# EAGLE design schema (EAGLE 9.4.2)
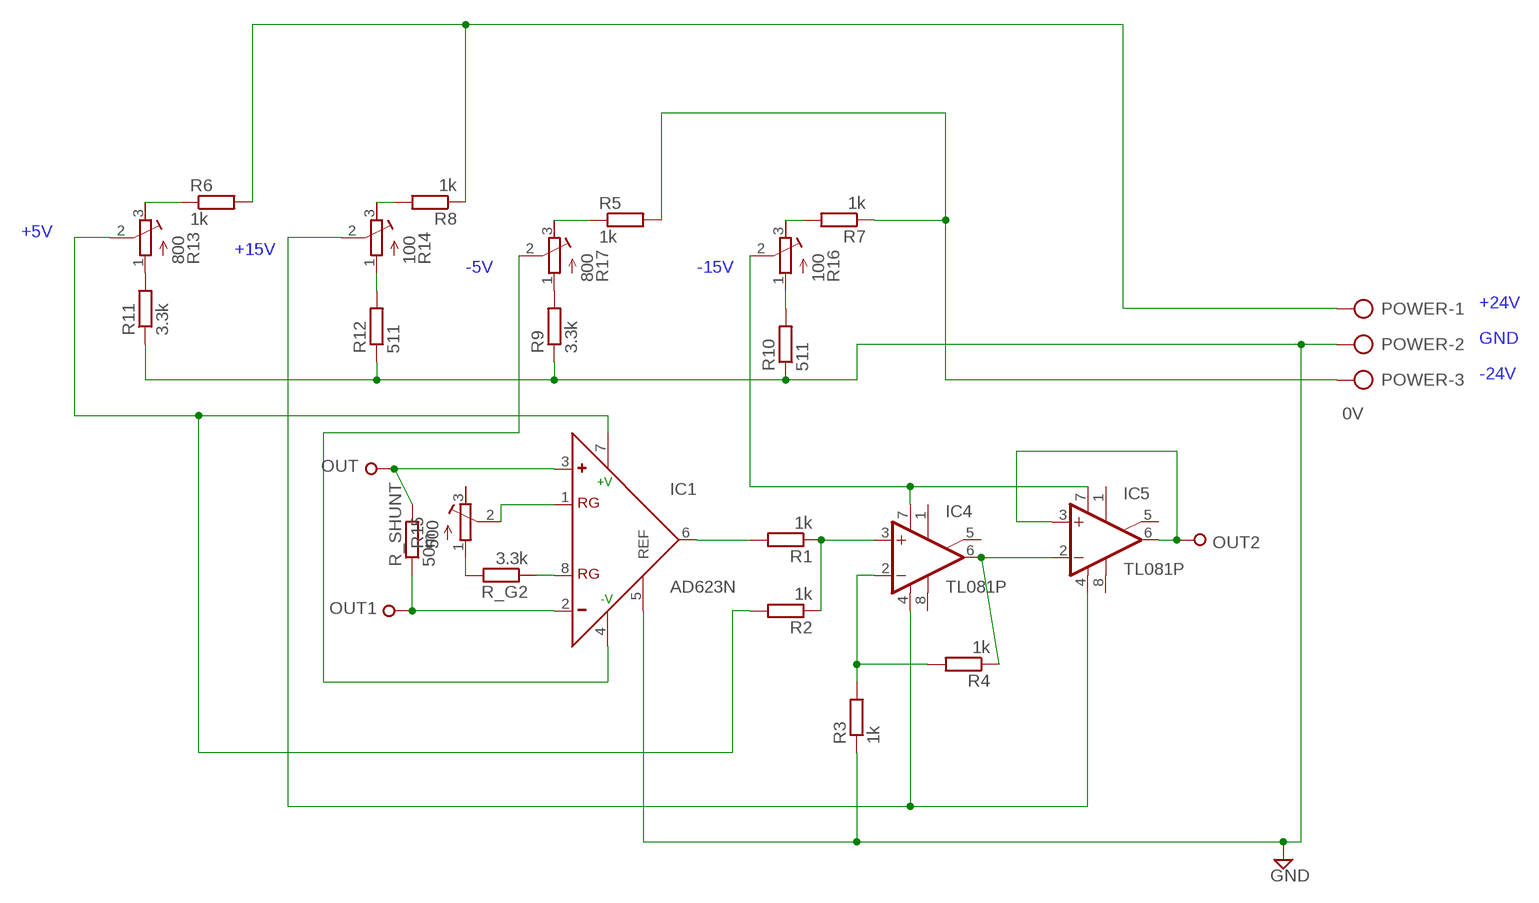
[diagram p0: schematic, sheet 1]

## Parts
IC1  AD623N  [DIL08]
IC4  TL081P  [DIL08]
IC5  TL081P  [DIL08]
OUT  SPECIAL_DRILL_0.2500  [PAD_0.2500]
OUT1  SPECIAL_DRILL_0.2500  [PAD_0.2500]
OUT2  SPECIAL_DRILL_0.2500  [PAD_0.2500]
POWER  0V  AK500/3-H  [AK500/3-H]
R1  1k  R-EU_0411/15  [0411/15]
R2  1k  R-EU_0411/15  [0411/15]
R3  1k  R-EU_0411/15  [0411/15]
R4  1k  R-EU_0411/15  [0411/15]
R5  1k  R-EU_0411/15  [0411/15]
R6  1k  R-EU_0411/15  [0411/15]
R7  1k  R-EU_0411/15  [0411/15]
R8  1k  R-EU_0411/15  [0411/15]
R9  3.3k  R-EU_0411/15  [0411/15]
R10  511  R-EU_0411/15  [0411/15]
R11  3.3k  R-EU_0411/15  [0411/15]
R12  511  R-EU_0411/15  [0411/15]
R13  800  R-TRIMM64X  [RTRIM64X]
R14  100  R-TRIMM64X  [RTRIM64X]
R15  500  R-TRIMM64X  [RTRIM64X]
R16  100  R-TRIMM64X  [RTRIM64X]
R17  800  R-TRIMM64X  [RTRIM64X]
R_G2  3.3k  R-EU_0411/15  [0411/15]
R_SHUNT  50m  R-EU_0309/12  [0309/12]

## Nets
GND: IC1.5(REF) POWER.2 R3.1 R9.1 R10.1 R11.1 R12.1
N$1: IC1.6(OUT) R1.2
N$2: IC4.2(-IN) R3.2 R4.2
N$3: IC4.3(+IN) R1.1 R2.1
N$4: IC4.6(OUT) IC5.2(-IN) R4.1
N$5: R15.1(A) R_G2.2
N$6: IC1.1(RG) R15.2(S)
N$7: IC1.8(RG) R_G2.1
N$8: IC1.2(-) OUT1.1 R_SHUNT.1
N$9: IC1.3(+) OUT.1 R_SHUNT.2
N$10: IC5.3(+IN) IC5.6(OUT) OUT2.1
N$11: R7.2 R16.3(E)
N$12: R5.1 R17.3(E)
N$13: R9.2 R17.1(A)
N$14: R10.2 R16.1(A)
N$15: R8.2 R14.3(E)
N$16: R6.1 R13.3(E)
N$17: R11.2 R13.1(A)
N$18: R12.2 R14.1(A)
N$19: POWER.1 R6.2 R8.1
N$20: POWER.3 R5.2 R7.1
N$22: IC4.7(V+) IC5.7(V+) R16.2(S)
N$23: IC1.4(-V) R17.2(S)
N$24: IC4.4(V-) IC5.4(V-) R14.2(S)
N$25: IC1.7(+V) R2.2 R13.2(S)
Unconnected: IC4.1(ON1) IC4.5(ON2) IC4.8(OPT) IC5.1(ON1) IC5.5(ON2) IC5.8(OPT) R15.3(E)

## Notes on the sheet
- +5V
- +15V
- -5V | -15V
- +24V
- GND
- -24V

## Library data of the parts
IC1 = analog-devices:AD623: Single-Supply, Rail-to-Rail, Low Cost Instrumentation Amplifier Source: http://www.analog.com/static/imported-files/data_sheets/AD623.pdf; MF: ALTERA CORPORATION; MPN: AD623ANZ; OC_FARNELL: 9603700; OC_NEWARK: 59K4402
IC4 IC5 = linear:TL081: OP AMP
OUT OUT1 OUT2 = special-drill:SPECIAL_DRILL_: Special drills
POWER = con-ptr500:AK500/3-H: CONNECTOR Aug. 2004 / PTR Meßtechnik: Die Bezeichnung der Serie AK505 wurde geändert. Es handelt sich hierbei um AK500 in horizontaler Ausführung.; OC_FARNELL: unknown; OC_NEWARK: unknown
R1-R12 R_G2 R_SHUNT = rcl:R-EU_: RESISTOR, European symbol; SPICEPREFIX: R
R13-R17 = rcl:R-TRIMM: Trimm resistor; SPICEMODEL: X; SPICEPREFIXL: POT

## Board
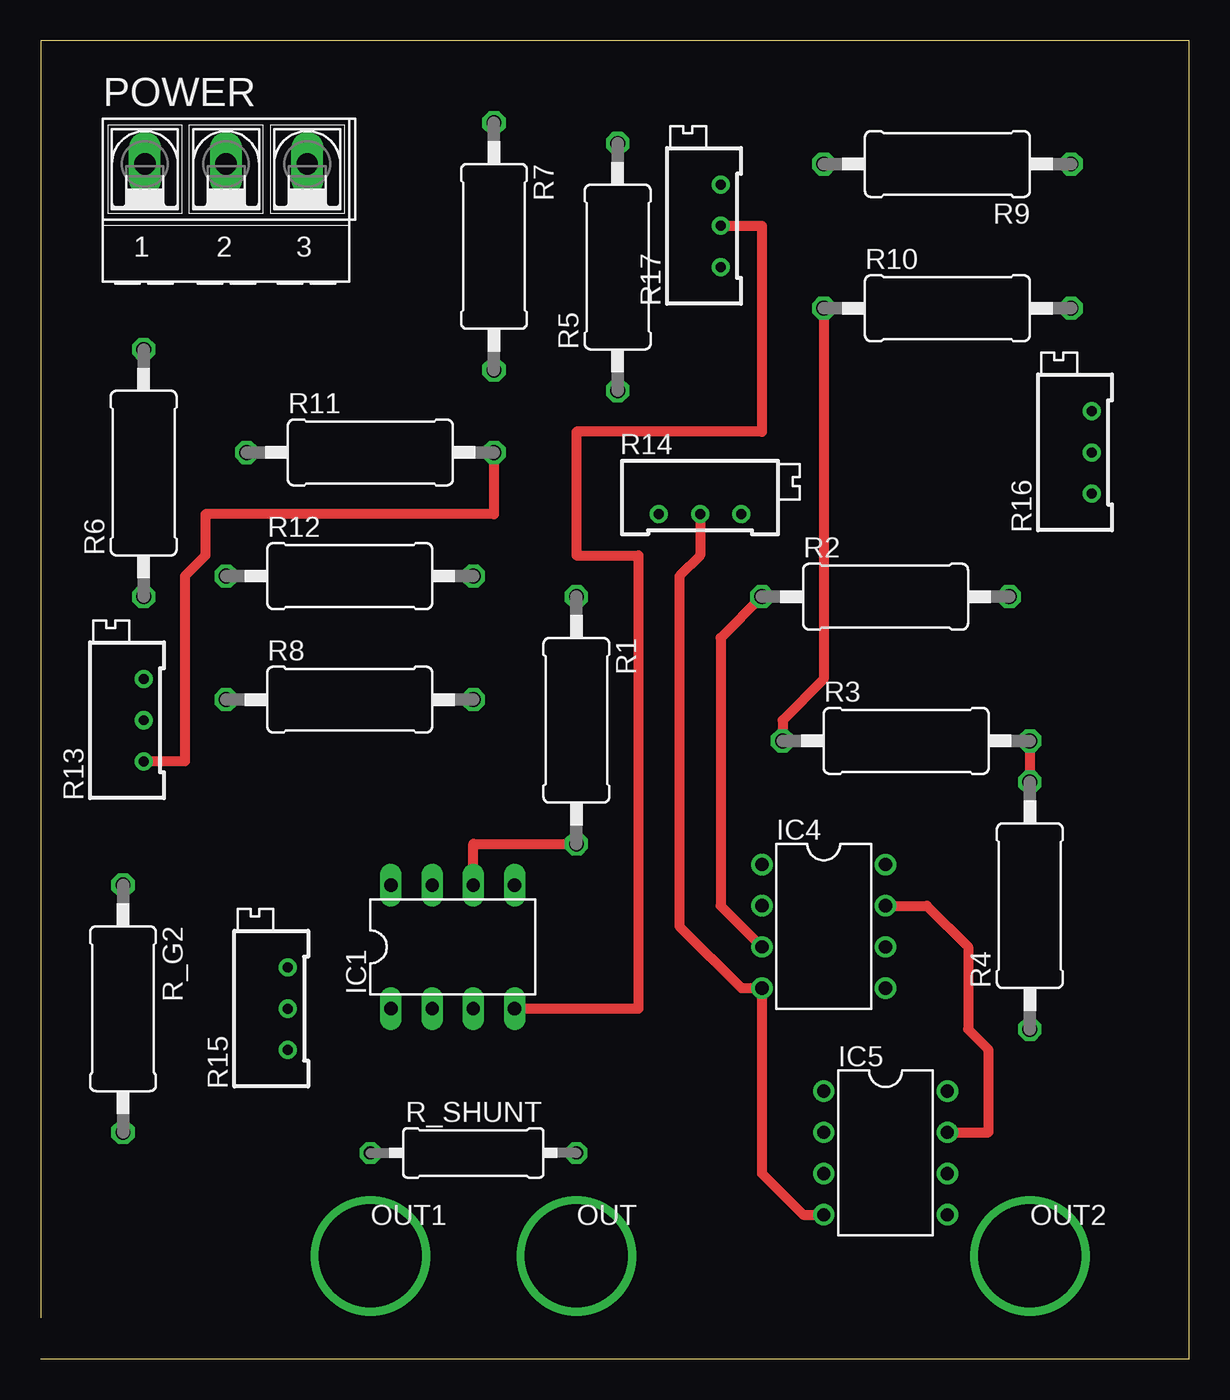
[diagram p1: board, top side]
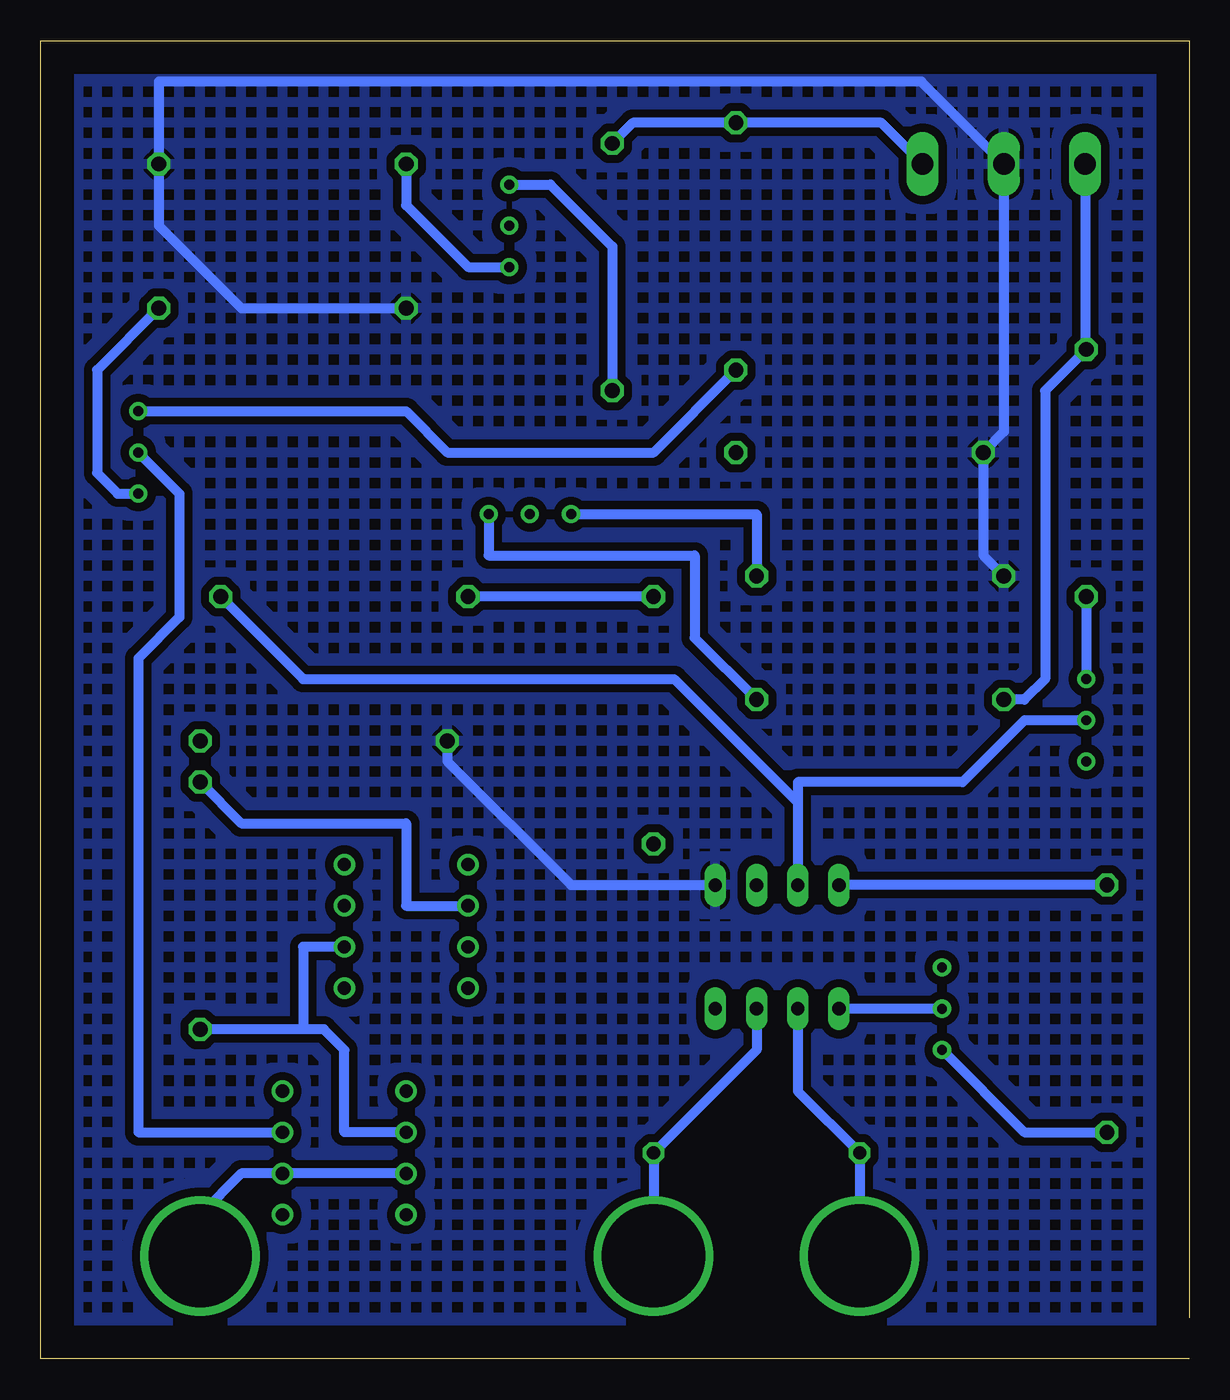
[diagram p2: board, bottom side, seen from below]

Size 70.79 x 81.27 mm. Coordinates in mm from the lower left corner, seen from the top.
Outline: 0,0 70.79,0 70.79,81.27 0,81.27 0,2.54
Copper layers (1*16): Top 0.035mm / dielectric 1.5mm / Bottom 0.035mm
Design rules "LBMS-ENIB": minimum track width 24mil, minimum drill 10mil, track to track 20mil, track to pad 20mil, pad to pad 20mil, via to via 20mil, smd to smd 8mil, copper to edge 80mil, drill to drill 8mil, minimum pad ring 10mil, minimum via ring 20mil, stop-mask expansion 4mil, vias tented up to drill 0mil, thermal gap 10mil

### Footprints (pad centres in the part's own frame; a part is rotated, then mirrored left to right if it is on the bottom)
DIL08 = drill 0.813 long: 1 -3.81,-3.81; 2 -1.27,-3.81; 3 1.27,-3.81; 4 3.81,-3.81; 5 3.81,3.81; 6 1.27,3.81; 7 -1.27,3.81; 8 -3.81,3.81
DIL08' = drill 0.813 pad 1.27: 1 -3.81,-3.81; 2 -1.27,-3.81; 3 1.27,-3.81; 4 3.81,-3.81; 5 3.81,3.81; 6 1.27,3.81; 7 -1.27,3.81; 8 -3.81,3.81
PAD_0.2500 = drill 6.35 pad 6.35: 1 0,0
AK500/3-H = drill 1.321 long: 1 -5.004,0; 2 0,0; 3 5.004,0
0411/15 = drill 0.914 octagon: 1 -7.62,0; 2 7.62,0
RTRIM64X = drill 0.61: 1 1.27,-2.54; 2 1.27,0; 3 1.27,2.54
0309/12 = drill 0.813 octagon: 1 -6.35,0; 2 6.35,0

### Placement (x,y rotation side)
IC1  25.4,25.4 0 top
IC4  TL081P  [DIL08']  48.26,26.67 270 top
IC5  TL081P  [DIL08']  52.07,12.7 270 top
OUT  33.02,6.35 0 top
OUT1  20.32,6.35 0 top
OUT2  60.96,6.35 0 top
POWER  11.43,73.66 0 top
R1  33.02,39.37 270 top
R2  52.07,46.99 0 top
R3  53.34,38.1 0 top
R4  60.96,27.94 90 top
R5  35.56,67.31 90 top
R6  6.35,54.61 90 top
R7  27.94,68.58 270 top
R8  19.05,40.64 0 top
R9  55.88,73.66 180 top
R10  55.88,64.77 0 top
R11  20.32,55.88 0 top
R12  19.05,48.26 0 top
R13  5.08,39.37 0 top
R14  40.64,53.34 270 top
R15  13.97,21.59 0 top
R16  63.5,55.88 0 top
R17  40.64,69.85 0 top
R_G2  5.08,21.59 270 top
R_SHUNT  26.67,12.7 0 top

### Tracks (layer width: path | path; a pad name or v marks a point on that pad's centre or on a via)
GND
  Top 0.61: R10.1 48.26,41.91 45.72,39.37 R3.1
  Bottom 0.61: R10.1 58.42,64.77 63.5,69.85 R9.1 63.5,78.74 16.51,78.74 POWER.2 11.43,57.15 R11.1 12.7,49.53 R12.1 | R3.1 45.72,36.83 38.1,29.21 IC1.5
  pour Bottom (hatched): 0,81.28 69.85,81.28 69.85,1.27 0,1.27
N$1
  Top 0.61: IC1.6 26.67,31.75 R1.2
N$2
  Top 0.61: R3.2 R4.2
  Bottom 0.61: R4.2 58.42,33.02 48.26,33.02 48.26,27.94 IC4.2
N$3
  Top 0.61: R2.1 41.91,44.45 41.91,27.94 IC4.3
  Bottom 0.61: R1.1 R2.1
N$4
  Bottom 0.61: IC5.2 52.07,13.97 52.07,19.05 53.34,20.32 54.61,20.32 | 54.61,20.32 R4.1 | IC4.6 54.61,25.4 54.61,20.32
N$5
  Bottom 0.61: R15.1 10.16,13.97 R_G2.2
N$6
  Bottom 0.61: R15.2 IC1.1
N$7
  Bottom 0.61: R_G2.1 IC1.8
N$8
  Bottom 0.61: IC1.2 24.13,16.51 R_SHUNT.1 OUT1.1
N$9
  Bottom 0.61: IC1.3 26.67,19.05 R_SHUNT.2 OUT.1
N$10
  Bottom 0.61: IC5.3 IC5.6 58.42,11.43 60.96,8.89 OUT2.1
N$11
  Bottom 0.61: R7.2 33.02,55.88 45.72,55.88 48.26,58.42 R16.3
N$12
  Bottom 0.61: R17.3 39.37,72.39 35.56,68.58 R5.1
N$13
  Bottom 0.61: R9.2 48.26,71.12 44.45,67.31 R17.1
N$14
  Bottom 0.61: R10.2 67.31,60.96 67.31,54.61 66.04,53.34 R16.1
N$15
  Bottom 0.61: R14.3 43.18,49.53 30.48,49.53 30.48,44.45 R8.2
N$16
  Bottom 0.61: R6.1 R13.3
N$17
  Top 0.61: R11.2 27.94,52.07 10.16,52.07 10.16,49.53 8.89,48.26 8.89,36.83 R13.1
N$18
  Bottom 0.61: R14.1 26.67,52.07 R12.2
N$19
  Bottom 0.61: POWER.1 6.43,62.31 R6.2 8.89,59.69 8.89,41.91 10.16,40.64 R8.1
N$20
  Bottom 0.61: POWER.3 18.97,76.2 R7.1 34.29,76.2 R5.2
N$22
  Top 0.61: IC4.7 54.61,27.94 57.15,25.4 57.15,20.32 58.42,19.05 58.42,13.97 IC5.7
  Bottom 0.61: R16.2 62.23,53.34 62.23,45.72 64.77,43.18 64.77,13.97 IC5.7
N$23
  Top 0.61: R17.2 44.45,69.85 44.45,57.15 33.02,57.15 33.02,49.53 36.83,49.53 36.83,21.59 IC1.4
N$24
  Top 0.61: R14.2 40.64,49.53 39.37,48.26 39.37,26.67 43.18,22.86 IC4.4 44.45,11.43 46.99,8.89 IC5.4
N$25
  Bottom 0.61: R13.2 10.16,39.37 13.97,35.56 24.13,35.56 24.13,34.29 | 24.13,34.29 IC1.7 | R2.2 54.61,41.91 31.75,41.91 24.13,34.29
